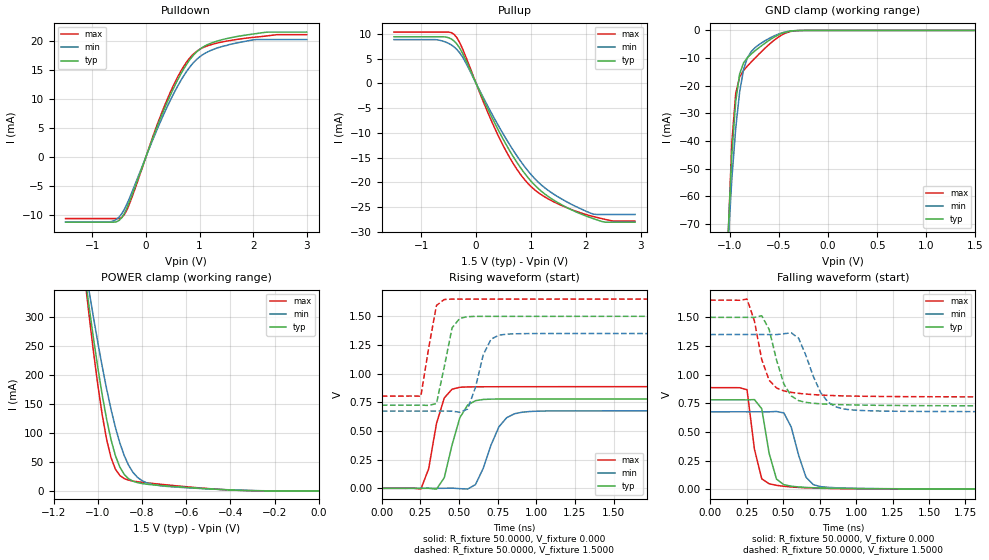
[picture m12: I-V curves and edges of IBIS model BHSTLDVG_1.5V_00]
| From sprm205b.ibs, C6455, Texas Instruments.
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|   Model BHSTLDVG_1.5V_00
[Model]   BHSTLDVG_1.5V_00
Model_type   I/O
Polarity   Non-Inverting
Enable   Active-Low
Vinl =   0.6500V
Vinh =   0.8500V
Vmeas =   0.7500V
Cref =   5.0000pF
Rref =  50.0000
Vref =   0.7500V
C_comp   1.2525pF   1.1880pF   1.2900pF
[Temperature Range]   25.0000   0.1250k   -40.0000
[Pullup Reference]   1.5000V   1.3500V   1.6500V
[Pulldown Reference]   0.000V   0.000V   0.000V
[POWER Clamp Reference]   1.5000V   1.3500V   1.6500V
[GND Clamp Reference]   0.000V   0.000V   0.000V
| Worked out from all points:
|   slope of the pulldown table from 0 to 0.225 V, typ, clamps not added: 40.4 ohm
|   slope of the pullup table from 0 to 0.225 V, typ, clamps not added: 41.4 ohm
|   GND clamp passes 1 mA (typ) near -0.47 V on its own axis
|   POWER clamp passes 1 mA (typ) near -0.35 V on its own axis
|   rising waveform, R_fixture 50.0000, V_fixture 0.000: 20-80 % time 93.3ps typ, 118ps min, 82.2ps max; typ from 0 V to 0.78 V
|   rising waveform, R_fixture 50.0000, V_fixture 1.5000: 20-80 % time 70.6ps typ, 87.9ps min, 65.1ps max; typ from 0.725 V to 1.5 V
|   falling waveform, R_fixture 50.0000, V_fixture 0.000: 20-80 % time 75.6ps typ, 92.5ps min, 68.5ps max; typ from 0.78 V to 0 V
|   falling waveform, R_fixture 50.0000, V_fixture 1.5000: 20-80 % time 110ps typ, 137ps min, 98ps max; typ from 1.5 V to 0.726 V
[Pulldown]
| voltage   I(typ)   I(min)   I(max)
-1.5V     -11.28mA   -11.23mA   -10.66mA
-600mV    -11.28mA   -11.04mA   NA
-500mV    -10.96mA   -10.38mA   -10.66mA
-400mV    -9.717mA   -9.005mA   -9.931mA
-300mV    -7.562mA   -6.965mA   -7.926mA
200mV     4.985mA    4.546mA    5.302mA
450mV     10.54mA    9.661mA    11.04mA
700mV     15.09mA    13.91mA    15.54mA
950mV     18.14mA    16.84mA    18.22mA
1.3V      19.89mA    18.68mA    19.57mA
1.9V      21.05mA    20.01mA    20.51mA
3V        21.52mA    20.23mA    21.08mA
[Pullup]
| voltage   I(typ)   I(min)   I(max)
-1.5V     9.441mA    8.863mA    10.39mA
-650mV    9.441mA    8.691mA    NA
-400mV    8.559mA    7.361mA    9.901mA
-200mV    5.007mA    4.419mA    5.73mA
200mV     -4.857mA   -4.338mA   -5.539mA
500mV     -11.43mA   -10.35mA   -12.73mA
800mV     -16.9mA    -15.56mA   -18.27mA
1.1V      -20.92mA   -19.62mA   -21.82mA
1.5V      -24.19mA   -23mA      -24.42mA
2.1V      -27.22mA   -26.31mA   -26.83mA
2.35V     -28.09mA   NA         -27.52mA
2.9V      -28.09mA   -26.53mA   -27.88mA
[GND_clamp]
| voltage   I(typ)   I(min)   I(max)
-1.5V     -1.991A    -1.52A     -2.425A
-1.02V    -75.55mA   -78.66mA   -77.37mA
-980mV    -44.93mA   -53.82mA   -40.69mA
-940mV    -25.58mA   -35.3mA    -22.79mA
-900mV    -15.71mA   -22.17mA   -16.79mA
-860mV    -11.7mA    -14.08mA   -14.47mA
-820mV    -9.791mA   -9.793mA   -12.83mA
-780mV    -8.452mA   -7.539mA   -11.32mA
-700mV    -6.146mA   -5.053mA   -8.422mA
-500mV    -1.502mA   -1.249mA   -2.257mA
-340mV    -87.74uA   -108.1uA   -144.7uA
1.5V      52.23nA    35.19uA    41.21nA
[POWER_clamp]
| voltage   I(typ)   I(min)   I(max)
-1.5V     1.855A     1.604A     2.098A
-1.06V    376.9mA    393.7mA    372mA
-1.04V    319.5mA    346.2mA    305.1mA
-1.02V    264.7mA    300.3mA    241.8mA
-1V       213.2mA    256.4mA    183.4mA
-960mV    123.8mA    176.1mA    89.05mA
-940mV    88.38mA    140.7mA    57.5mA
-920mV    60.69mA    109.3mA    37.47mA
-880mV    28.35mA    60.73mA    21.23mA
-820mV    14.22mA    23.32mA    15.8mA
-740mV    10.13mA    10.22mA    12.42mA
0V        52.23nA    112.8nA    78.79nA
[Ramp]
| variable   typ   min   max
dV/dt_r   0.4679/92.2978p   0.4053/0.1171n   0.5318/86.2567p
dV/dt_f   0.4647/0.1087n   0.4054/0.1358n   0.5075/96.9572p
R_load = 50.0000
[Rising Waveform]
R_fixture = 50.0000
V_fixture = 0.000
V_fixture_min = 0.000
V_fixture_max = 0.000
| time   V(typ)   V(min)   V(max)
0s        37.04uV    55.49uV    40.22uV
252.5ps   147.1uV    57.3uV     -6.503mV
303ps     1.11mV     63.28uV    169.9mV
353.5ps   -7.287mV   7.612uV    564mV
404ps     92.55mV    421.4uV    788.3mV
505.1ps   616.5mV    -3.044mV   881.1mV
606.1ps   764.1mV    32.83mV    885mV
757.6ps   778.3mV    535.7mV    885.6mV
909.1ps   778.9mV    663.6mV    885.8mV
5ns       779.9mV    675.5mV    886.4mV
[Rising Waveform]
R_fixture = 50.0000
V_fixture = 1.5000
V_fixture_min = 1.3500
V_fixture_max = 1.6500
| time   V(typ)   V(min)   V(max)
0s        725.1mV    673.5mV    803.7mV
252.5ps   725.3mV    673.5mV    802.7mV
353.5ps   738.9mV    673.4mV    1.595V
404ps     1.059V     674mV      1.646V
454.5ps   1.4V       672.8mV    1.65V
505.1ps   1.483V     663.3mV    1.649V
555.6ps   1.497V     691.4mV    1.649V
707.1ps   1.499V     1.301V     1.649V
808.1ps   1.499V     1.344V     1.649V
5ns       1.5V       1.35V      1.65V
[Falling Waveform]
R_fixture = 50.0000
V_fixture = 0.000
V_fixture_min = 0.000
V_fixture_max = 0.000
| time   V(typ)   V(min)   V(max)
0s        779.9mV    675.7mV    886.4mV
252.5ps   779.6mV    675.7mV    868mV
303ps     782.1mV    675.7mV    350.7mV
353.5ps   701.7mV    675.7mV    89.93mV
404ps     313.1mV    675.2mV    47.57mV
454.5ps   87.91mV    678.3mV    33.78mV
555.6ps   26.16mV    542.3mV    19.51mV
656.6ps   15.38mV    104.7mV    12.21mV
757.6ps   10.46mV    22.28mV    8.141mV
5ns       361.5uV    590.4uV    289.3uV
[Falling Waveform]
R_fixture = 50.0000
V_fixture = 1.5000
V_fixture_min = 1.3500
V_fixture_max = 1.6500
| time   V(typ)   V(min)   V(max)
0s        1.5V       1.35V      1.65V
252.5ps   1.5V       1.35V      1.659V
353.5ps   1.514V     1.35V      1.131V
404ps     1.394V     1.349V     950.8mV
505.1ps   917.7mV    1.357V     858.1mV
555.6ps   814.1mV    1.365V     845.1mV
606.1ps   773.1mV    1.318V     836.6mV
757.6ps   745.1mV    841.6mV    821.8mV
959.6ps   735.8mV    693mV      813.1mV
5ns       725.6mV    674.3mV    804.1mV
